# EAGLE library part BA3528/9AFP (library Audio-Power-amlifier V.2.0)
Pre / power amplifier and motor governor for 3V headphone stereos
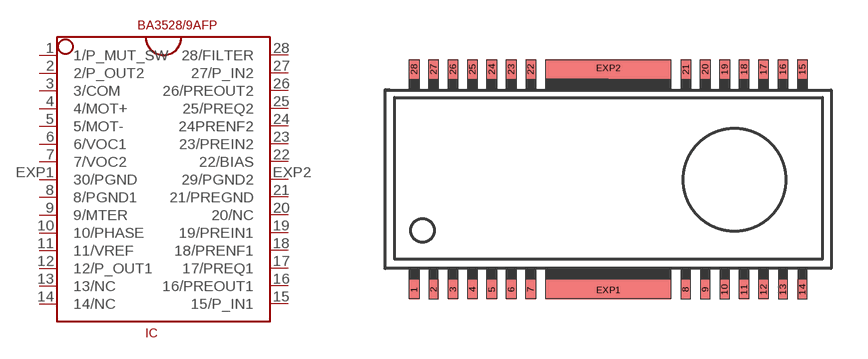
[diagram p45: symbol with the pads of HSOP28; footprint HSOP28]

Designator prefix IC

## BA3528/9AFP  [HSOP28]
1  1/P_MUT_SW
2  2/P_OUT2  out
3  3/COM
4  4/MOT+  out
5  5/MOT-  out
6  6/VOC1  pwr
7  7/VOC2  pwr
8  8/PGND1  pwr
9  9/MTER
10  10/PHASE
11  11/VREF
12  12/P_OUT1  out
13  13/NC  nc
14  14/NC  nc
15  15/P_IN1  in
16  16/PREOUT1  out
17  17/PREQ1
18  18/PRENF1
19  19/PREIN1  in
20  20/NC  nc
21  21/PREGND  pwr
22  22/BIAS
23  23/PREIN2  in
24  24PRENF2
25  25/PREQ2
26  26/PREOUT2  out
27  27/P_IN2  in
28  28/FILTER
EXP1  30/PGND  pwr
EXP2  29/PGND2  pwr

## Footprint HSOP28 (pad centres in mm)
smd 0.406 x 0.813: 1 -8,-4.545; 2 -7.2,-4.545; 3 -6.4,-4.545; 4 -5.6,-4.545; 5 -4.8,-4.545; 6 -4,-4.545; 7 -3.2,-4.545; 8 3.19,-4.545; 9 4,-4.545; 10 4.795,-4.545; 11 5.6,-4.545; 12 6.4,-4.545; 13 7.2,-4.545; 14 8,-4.545; 15 8,4.545; 16 7.2,4.545; 17 6.4,4.545; 18 5.6,4.545; 19 4.8,4.545; 20 4,4.545; 21 3.2,4.545; 22 -3.2,4.545; 23 -4,4.545; 24 -4.8,4.545; 25 -5.6,4.545; 26 -6.4,4.545; 27 -7.2,4.545; 28 -8,4.545
smd 0.813 x 0.406: EXP1 0.005,-4.57; EXP2 0,4.595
